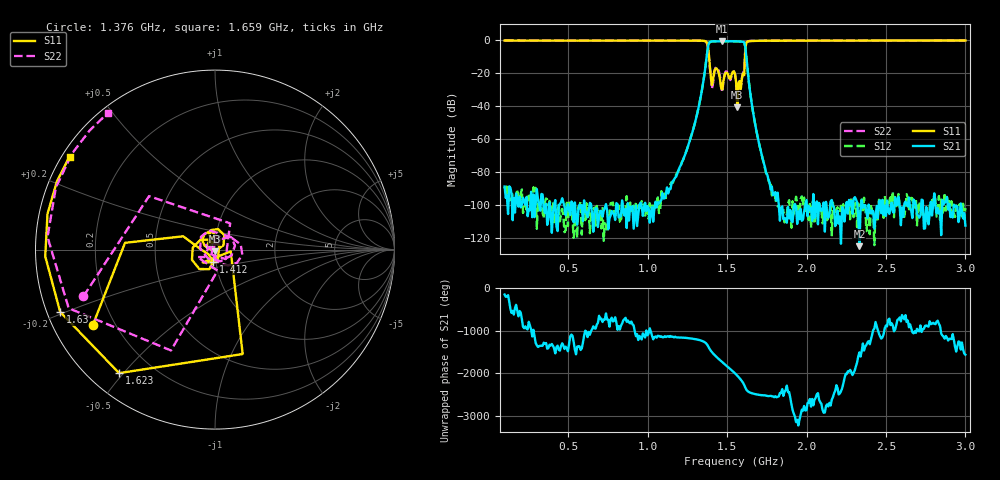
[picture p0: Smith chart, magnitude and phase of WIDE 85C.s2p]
!Agilent Technologies,E8364B,MY43040699,A.07.50.67
!Agilent E8364B: A.07.50.67
!Date: Wednesday, June 25, 2025 06:03:48
!Correction: S11(Full 2 Port(1,2))
!S21(Full 2 Port(1,2))
!S12(Full 2 Port(1,2))
!S22(Full 2 Port(1,2))
!S2P File: Measurements: S11, S21, S12, S22:
# Hz S  dB  R 50
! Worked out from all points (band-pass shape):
!   401 points, 100 MHz to 3 GHz, reference 50 ohm
!   highest |S21| = -0.49 dB at 1.47 GHz (marker M1); lowest = -124.9 dB at 2.333 GHz (marker M2)
!   |S21| within 3 dB of the highest: 1.382 GHz to 1.614 GHz (232.3 MHz wide, 15.5 % of centre)
!   lowest |S11| = -40.7 dB at 1.565 GHz (marker M3), VSWR 1.02, Z = 49.9 - j0.92 ohm
!   |S11| at or under -10 dB: 1.387 GHz to 1.613 GHz (226.1 MHz wide, 15.1 % of centre)
!   |S22| runs from -39.0 to 0.0 dB; largest |S21 - S12| = 0.001
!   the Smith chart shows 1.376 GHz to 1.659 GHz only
!   S11 on the Smith chart (normalised r, x): 1.376 GHz: 0.12, -0.28; 1.412 GHz: 0.97, -0.13; 1.623 GHz: 0.09, -0.49; 1.63 GHz: 0.04, -0.19; 1.659 GHz: 0.02, +0.29
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1e8  -0.07 168.7  -88.69 -148.0  -88.74 -100.5  -0.04 168.6
5.8575e8  -0.14 112.1  -99.98 29.4  -117.87 0.1  -0.11 111.9
1.0715e9  -0.09 45.3  -98.93 -40.9  -104.79 -78.9  -0.09 47.6
1.2165e9  -0.07 10.7  -73.83 -78.6  -73.54 -79.0  -0.08 15.7
1.318e9  -0.12 -41.0  -41.98 -129.2  -41.95 -129.1  -0.12 -32.6
1.376e9  -1.96 -148.4  -6.70 109.9  -6.70 109.9  -2.18 -160.4
1.41225e9  -23.38 -98.3  -0.59 -92.7  -0.59 -92.7  -25.65 83.5
1.44125e9  -18.10 175.0  -0.58 160.3  -0.59 160.4  -16.92 -31.0
1.47025e9  -29.74 157.0  -0.49 64.0  -0.49 64.0  -31.53 143.8
1.492e9  -19.64 124.3  -0.54 -5.8  -0.54 -5.7  -18.90 37.7
1.51375e9  -22.93 92.1  -0.51 -75.6  -0.52 -75.6  -22.80 -63.1
1.55e9  -20.36 57.4  -0.58 161.5  -0.58 161.5  -20.59 81.1
1.5645e9  -40.66 -95.7  -0.57 107.2  -0.58 107.2  -39.02 135.6
1.58625e9  -29.55 45.4  -0.68 15.2  -0.68 15.3  -28.51 162.1
1.6225e9  -1.20 -127.8  -11.23 133.1  -11.22 133.1  -1.13 -158.2
1.62975e9  -0.63 -158.1  -18.58 103.8  -18.58 103.8  -0.58 175.7
1.65875e9  -0.34 147.4  -40.61 51.2  -40.60 51.1  -0.30 128.2
1.753e9  -0.19 89.5  -81.38 -8.1  -82.13 -7.8  -0.16 76.6
2.03575e9  -0.10 33.2  -109.50 -79.7  -98.34 -83.7  -0.09 24.7
2.333e9  -0.08 1.2  -124.85 -65.4  -105.76 127.6  -0.08 -6.0
2.5215e9  -0.08 -15.5  -105.25 5.9  -97.95 -62.5  -0.07 -22.2
3e9  -0.07 -52.4  -112.41 -120.8  -101.70 75.8  -0.07 -58.5
